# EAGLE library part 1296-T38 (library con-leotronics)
1.27mm SINGLE ROW FEMALE SOCKET Source: http://www.leotronics.co.uk/Conexcon/Data%20Sheets/sec.%20A/1296ing.pdf
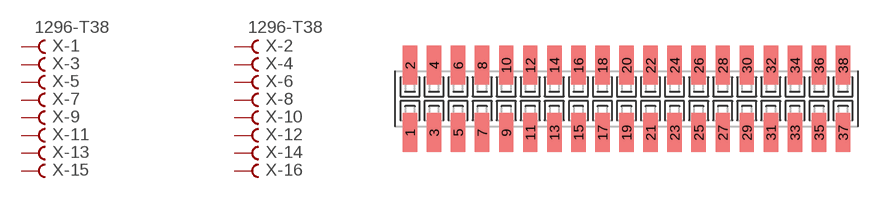
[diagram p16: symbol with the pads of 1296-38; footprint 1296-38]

Designator prefix X; gates -1=FVAL -2=FVAL -3=F -4=F -5=F -6=F -7=F -8=F -9=F -10=F -11=F -12=F -13=F -14=F -15=F -16=F -17=F -18=F -19=F -20=F -21=F -22=F -23=F -24=F -25=F -26=F -27=F -28=F -29=F -30=F -31=F -32=F -33=F -34=F -35=F -36=F -37=F -38=F

## 1296-T38 (OC_FARNELL: unknown; OC_NEWARK: unknown)  [1296-38]
1  -1:B  pas
2  -2:B  pas
3  -3:B  pas
4  -4:B  pas
5  -5:B  pas
6  -6:B  pas
7  -7:B  pas
8  -8:B  pas
9  -9:B  pas
10  -10:B  pas
11  -11:B  pas
12  -12:B  pas
13  -13:B  pas
14  -14:B  pas
15  -15:B  pas
16  -16:B  pas
17  -17:B  pas
18  -18:B  pas
19  -19:B  pas
20  -20:B  pas
21  -21:B  pas
22  -22:B  pas
23  -23:B  pas
24  -24:B  pas
25  -25:B  pas
26  -26:B  pas
27  -27:B  pas
28  -28:B  pas
29  -29:B  pas
30  -30:B  pas
31  -31:B  pas
32  -32:B  pas
33  -33:B  pas
34  -34:B  pas
35  -35:B  pas
36  -36:B  pas
37  -37:B  pas
38  -38:B  pas

## Footprint 1296-38 (pad centres in mm)
1.27mm SINGLE ROW FEMALE SOCKET Source: http://www.leotronics.co.uk/Conexcon/Data%20Sheets/sec.%20A/1296ing.pdf
smd 0.76 x 2.05: 1 -11.43,-1.78; 2 -11.43,1.78; 3 -10.16,-1.78; 4 -10.16,1.78; 5 -8.89,-1.78; 6 -8.89,1.78; 7 -7.62,-1.78; 8 -7.62,1.78; 9 -6.35,-1.78; 10 -6.35,1.78; 11 -5.08,-1.78; 12 -5.08,1.78; 13 -3.81,-1.78; 14 -3.81,1.78; 15 -2.54,-1.78; 16 -2.54,1.78; 17 -1.27,-1.78; 18 -1.27,1.78; 19 0,-1.78; 20 0,1.78; 21 1.27,-1.78; 22 1.27,1.78; 23 2.54,-1.78; 24 2.54,1.78; 25 3.81,-1.78; 26 3.81,1.78; 27 5.08,-1.78; 28 5.08,1.78; 29 6.35,-1.78; 30 6.35,1.78; 31 7.62,-1.78; 32 7.62,1.78; 33 8.89,-1.78; 34 8.89,1.78; 35 10.16,-1.78; 36 10.16,1.78; 37 11.43,-1.78; 38 11.43,1.78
